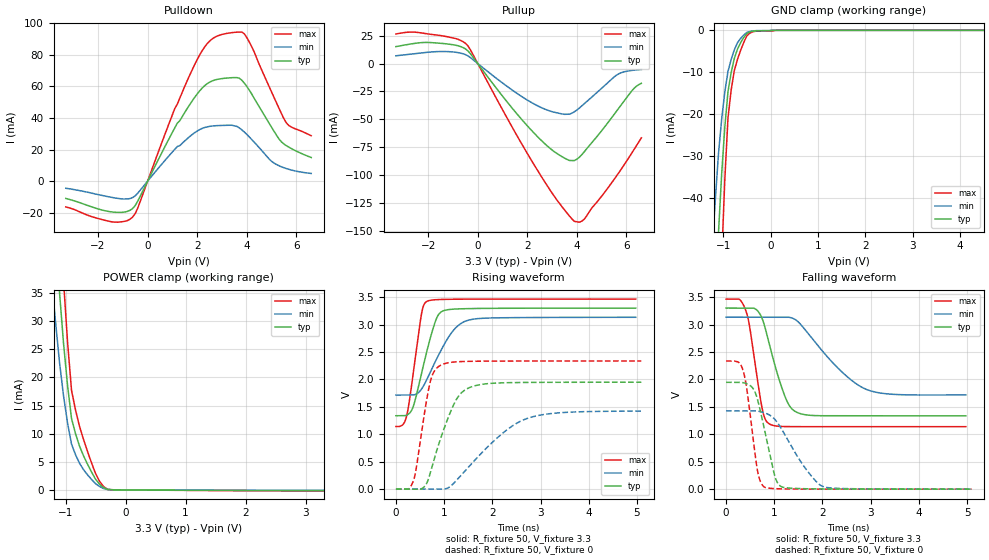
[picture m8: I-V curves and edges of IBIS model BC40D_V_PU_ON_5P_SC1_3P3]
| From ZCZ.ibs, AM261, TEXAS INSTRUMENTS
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[Model]   BC40D_V_PU_ON_5P_SC1_3P3
Model_type   I/O
Polarity   Non-Inverting
Enable   Active-Low
Vinl =  0.8V
Vinh =  2V
Cref =  15pF
Rref =  100.0000M
Vref =  0V
Vmeas =  1.65
C_comp   2.059994p   1.862014p   2.067327p
|[Input load] weak_pu_on
|[Output drive] slow
|[supplytol] 5
|[temp] ind
[Model Spec]
Vinl   0.8V   0.8V   0.8V
Vinh   2V   2V   2V
[Temperature Range]   25   125   -40
[Voltage Range]   3.3   3.135   3.465
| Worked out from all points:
|   slope of the pulldown table from 0 to 0.495 V, typ, clamps not added: 31.8 ohm
|   slope of the pullup table from 0 to 0.495 V, typ, clamps not added: 33.8 ohm
|   GND clamp passes 1 mA (typ) near -0.52 V on its own axis
|   POWER clamp passes 1 mA (typ) near -0.43 V on its own axis
|   rising waveform, R_fixture 50, V_fixture 3.3: 20-80 % time 333ps typ, 511ps min, 217ps max; typ from 1.34 V to 3.3 V
|   rising waveform, R_fixture 50, V_fixture 0: 20-80 % time 466ps typ, 1.01ns min, 251ps max; typ from 0 V to 1.95 V
|   falling waveform, R_fixture 50, V_fixture 3.3: 20-80 % time 385ps typ, 889ps min, 239ps max; typ from 3.3 V to 1.34 V
|   falling waveform, R_fixture 50, V_fixture 0: 20-80 % time 293ps typ, 607ps min, 204ps max; typ from 1.95 V to 0.002 V
| Nom Voltages:
|   VDD=1.1, VDDS=3.3, VDDS18=1.8, ESD_BIASFET=0, VSS=0, VSSS=0
| Min Voltages:
|   VDD=1.045, VDDS=3.135, VDDS18=1.71, ESD_BIASFET=0, VSS=0, VSSS=0
| Max Voltages:
|   VDD=1.16, VDDS=3.465, VDDS18=1.89, ESD_BIASFET=0, VSS=0, VSSS=0
[POWER_clamp]
|   voltage   I(typ)   I(min)   I(max)
-3.3V     446.9mA    437.1mA    604mA
-1.233V   56.55mA    37.5mA     80.28mA
-1.167V   45.63mA    29.89mA    65.07mA
-1.1V     35.1mA     22.65mA    50.26mA
-1.033V   26.08mA    16.75mA    37.2mA
-966.7mV  18.62mA    11.92mA    26.34mA
-900mV    12.7mA     8.144mA    17.7mA
-833.3mV  10mA       6.261mA    14.22mA
-766.7mV  7.795mA    4.75mA     11.31mA
-566.7mV  3.199mA    1.871mA    4.824mA
-366.7mV  433.5uA    268.9uA    617.1uA
3.3V      -100.3uA   -54.66uA   -173.1uA
[Pulldown]
|   voltage   I(typ)   I(min)   I(max)
-3.3V     -10.93mA   -4.474mA   -16.27mA
-1.4V     -19.53mA   -10.38mA   -25.83mA
-600mV    -17.23mA   -10.34mA   -22.61mA
1.2V      36.72mA    21.93mA    48.77mA
1.9V      53.02mA    30.66mA    73.76mA
2.4V      61.61mA    34.34mA    86.89mA
3V        64.86mA    35.24mA    92.76mA
3.6V      65.51mA    34.65mA    94.24mA
3.9V      62.01mA    31.1mA     93.16mA
5V        34.1mA     12.57mA    56.41mA
5.6V      22.42mA    7.958mA    36.79mA
6.6V      14.97mA    4.886mA    28.74mA
[Pullup]
|   voltage   I(typ)   I(min)   I(max)
-3.3V     15.12mA    6.907mA    26.36mA
-1.9V     18.73mA    10.27mA    26.12mA
-900mV    16.4mA     10.09mA    22.38mA
-400mV    11.39mA    6.888mA    15.9mA
1.3V      -37.44mA   -22.28mA   -53.31mA
2.4V      -65.08mA   -37.64mA   -95.03mA
3.3V      -81.9mA    -44.62mA   -125mA
3.9V      -86.71mA   -43.1mA    -141mA
4.3V      -78.82mA   -35.86mA   -139.1mA
5.6V      -42.54mA   -10.35mA   -100.4mA
6.3V      -22.29mA   -5.95mA    -77mA
6.6V      -17.71mA   -5.359mA   -66.44mA
[GND_clamp]
|   voltage   I(typ)   I(min)   I(max)
-3.3V     -787.2mA   -627.7mA   -1.235A
-1.233V   -85.67mA   -52.14mA   -138.8mA
-1.167V   -66.48mA   -40.37mA   -107.8mA
-1.1V     -48.26mA   -29.38mA   -78.01mA
-1.033V   -34.3mA    -21.2mA    -54.61mA
-966.7mV  -23.1mA    -14.68mA   -35.59mA
-900mV    -14.66mA   -9.807mA   -20.94mA
-833.3mV  -10.12mA   -6.96mA    -14.29mA
-700mV    -4.501mA   -2.971mA   -6.963mA
-500mV    -717.7uA   -493.4uA   -1.262mA
100mV     0A         0A         0A
6.6V      0A         0A         0A
[Ramp]
| variable   typ   min   max
dV/dt_f  1.1795006/0.38538225n 0.85573709/0.89559792n  1.3970808/0.23966865n
dV/dt_r  1.1738038/0.46664243n 0.86214199/1.0172278n  1.4060326/0.25228723n
R_load = 50
[Rising Waveform]
R_fixture = 50
V_fixture = 3.3
V_fixture_min = 3.135
V_fixture_max = 3.465
|   time   V(typ)   V(min)   V(max)
0s        1.338V     1.715V     1.141V
139.3ps   1.338V     1.715V     1.172V
221.2ps   1.349V     1.715V     1.327V
358.8ps   1.505V     1.716V     2.109V
529.7ps   2.102V     1.823V     3.191V
640.2ps   2.509V     1.996V     3.422V
905.9ps   3.206V     2.481V     3.457V
1.197ns   3.282V     2.899V     3.462V
1.482ns   3.29V      3.074V     3.463V
4.974ns   3.3V       3.133V     3.465V
[Rising Waveform]
R_fixture = 50
V_fixture = 0
V_fixture_min = 0
V_fixture_max = 0
|   time   V(typ)   V(min)   V(max)
0s        0V         2.1mV      3.387mV
263ps     0V         2.1mV      3.387mV
360.8ps   0V         2.1mV      149mV
574.7ps   33.49mV    2.1mV      1.285V
703.7ps   267.2mV    2.1mV      1.927V
932.1ps   936.8mV    2.1mV      2.261V
1.275ns   1.665V     178mV      2.322V
1.623ns   1.881V     515.3mV    2.331V
2.782ns   1.946V     1.306V     2.336V
5.091ns   1.949V     1.423V     2.336V
[Falling Waveform]
R_fixture = 50
V_fixture = 3.3
V_fixture_min = 3.135
V_fixture_max = 3.465
|   time   V(typ)   V(min)   V(max)
0s        3.3V       3.134V     3.464V
277.3ps   3.3V       3.134V     3.457V
413.4ps   3.3V       3.134V     3.247V
752.8ps   3.102V     3.134V     1.456V
904.2ps   2.62V      3.134V     1.188V
1.248ns   1.635V     3.134V     1.142V
1.515ns   1.385V     3.033V     1.141V
2.314ns   1.339V     2.213V     1.14V
2.895ns   1.339V     1.825V     1.14V
4.974ns   1.338V     1.718V     1.14V
[Falling Waveform]
R_fixture = 50
V_fixture = 0
V_fixture_min = 0
V_fixture_max = 0
|   time   V(typ)   V(min)   V(max)
0s        1.948V     1.429V     2.335V
357ps     1.94V      1.429V     2.151V
437ps     1.919V     1.429V     1.789V
651.7ps   1.638V     1.424V     340.1mV
795.3ps   1.095V     1.393V     40.31mV
1.019ns   220.1mV    1.266V     11.06mV
1.177ns   38.3mV     1.06V      6.738mV
1.65ns    9.475mV    377.4mV    3.314mV
2.027ns   6.06mV     45.49mV    3.009mV
5.091ns   2.104mV    3.384mV    2.775mV
